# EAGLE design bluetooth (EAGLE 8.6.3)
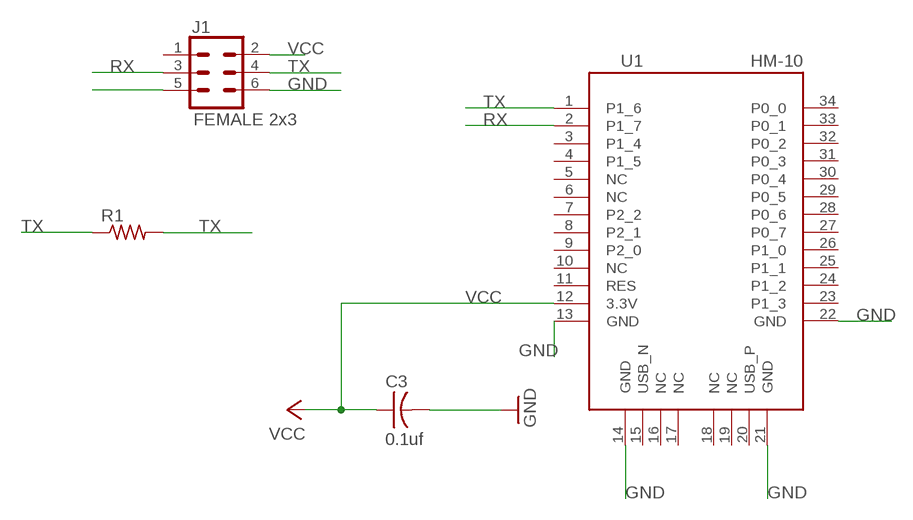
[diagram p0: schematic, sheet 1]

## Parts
C3  0.1uf  CAP-US1206FAB  [C1206FAB]
J1  FEMALE 2x3  CONN_03X2FEMALE  [2X3]
R1  RES-US1206FAB  [R1206FAB]
U1  HM-10  [HM-10]

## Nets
GND: C3.2 J1.6 U1.13(GND) U1.14(GND) U1.21(GND) U1.22(GND)
N$2: J1.5
RX: J1.3 U1.2(P1_7)
TX: J1.4 R1.1 R1.2 U1.1(P1_6)
VCC: C3.1 J1.2 U1.12(3.3V)
Unconnected: J1.1 U1.3(P1_4) U1.4(P1_5) U1.5(NC) U1.6(NC) U1.7(P2_2) U1.8(P2_1) U1.9(P2_0) U1.10(NC) U1.11(RES) U1.15(USB_N) U1.16(NC) U1.17(NC) U1.18(NC) U1.19(NC) U1.20(USB_P) U1.23(P1_3) U1.24(P1_2) U1.25(P1_1) U1.26(P1_0) U1.27(P0_7) U1.28(P0_6) U1.29(P0_5) U1.30(P0_4) U1.31(P0_3) U1.32(P0_2) U1.33(P0_1) U1.34(P0_0)

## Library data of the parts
C3 = private:CAP-US
J1 = private:CONN_03X2: Multi connection point. Often used as Generic Header-pin footprint for 0.1 inch spaced/style header connections You can populate with any combo of single row headers, but if you'd like an exact match, check these: Header - 2x3 (Male, 0.1") (PRT-12807) Header - 2x3 (Female, 0.1") (PRT-13010) 2x3 Pin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; PROD_ID: CONN-11566
R1 = private:RES-US: Resistor (US Symbol)
U1 = private:HM-10

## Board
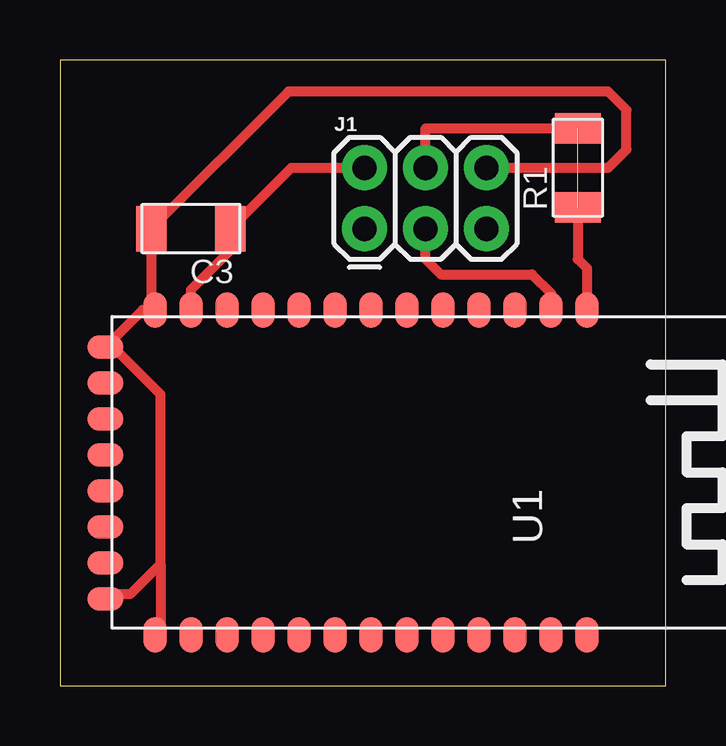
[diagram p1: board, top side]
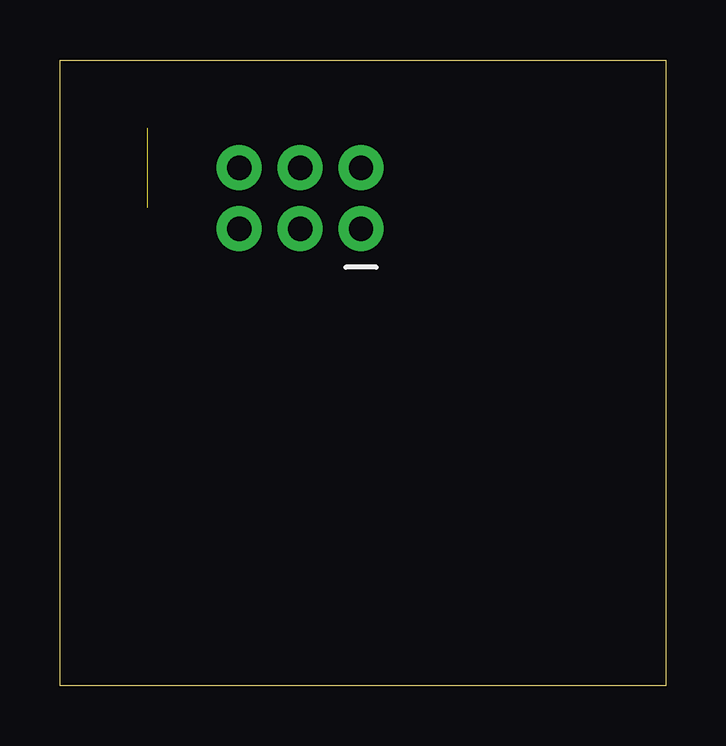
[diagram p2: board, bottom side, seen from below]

Size 25.25 x 26.09 mm. Coordinates in mm from the lower left corner, seen from the top.
Outline: 0,0 25.25,0 25.25,26.09 0,26.09 0,0
Copper layers (1*16): Top 0.035mm / dielectric 1.5mm / Bottom 0.035mm
Design rules "default *": minimum track width 15mil, minimum drill 0.79mm, track to track 0.4mm, track to pad 0.4mm, pad to pad 0.4mm, via to via 0.4mm, smd to smd 0.4mm, copper to edge 40mil, drill to drill 6mil, minimum pad ring 10mil, minimum via ring 8mil, stop-mask expansion 4mil, vias tented up to drill 0mil, thermal gap 10mil

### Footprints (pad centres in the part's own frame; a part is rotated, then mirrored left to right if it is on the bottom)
C1206FAB = smd 1.27 x 1.905: 1 -1.651,0; 2 1.651,0
2X3 = drill 1.016 pad 1.88: 1 0,0; 2 0,2.54; 3 2.54,0; 4 2.54,2.54; 5 5.08,0; 6 5.08,2.54
R1206FAB = smd 1.27 x 1.905: 1 -1.651,0; 2 1.651,0
HM-10 = smd 1.5 x 1: 1 -6.77,6.35; 2 -6.77,4.85; 3 -6.77,3.35; 4 -6.77,1.85; 5 -6.77,0.35; 6 -6.77,-1.15; 7 -6.77,-2.65; 8 -6.77,-4.15; 9 -6.77,-5.65; 10 -6.77,-7.15; 11 -6.77,-8.65; 12 -6.77,-10.15; 13 -6.77,-11.65; 22 6.77,-11.65; 23 6.77,-10.15; 24 6.77,-8.65; 25 6.77,-7.15; 26 6.77,-5.65; 27 6.77,-4.15; 28 6.77,-2.65; 29 6.77,-1.15; 30 6.77,0.35; 31 6.77,1.85; 32 6.77,3.35; 33 6.77,4.85; 34 6.77,6.35 | smd 1 x 1.5: 14 -5.23,-13.72; 15 -3.73,-13.72; 16 -2.23,-13.72; 17 -0.73,-13.72; 18 0.77,-13.72; 19 2.27,-13.72; 20 3.77,-13.72; 21 5.27,-13.72

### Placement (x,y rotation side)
C3  5.46,19.05 180 top
J1  12.7,19.05 0 top
R1  21.59,21.59 90 top
U1  15.62,8.89 270 top

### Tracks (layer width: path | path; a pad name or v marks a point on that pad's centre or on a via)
GND
  Top 0.406: 4.19,5.08 4.19,12.14 2.21,14.12 U1.14 3.44,15.66 U1.13 3.81,15.82 C3.2 9.53,24.77 22.86,24.77 23.62,24 23.62,22.35 22.86,21.59 J1.6 | 4.19,5.08 2.92,3.81 2.09,3.81 U1.21 | 4.19,5.08 4.19,2.34 U1.22
RX
  Top 0.406: U1.2 20.47,16.36 19.68,17.14 15.88,17.14 15.24,17.78 J1.3
TX  (1 unrouted)
  Top 0.406: U1.1 21.97,17.4 21.59,17.78 R1.1 | R1.2 15.24,23.24 J1.4
VCC
  Top 0.406: U1.12 5.46,16.51 7.11,18.16 C3.1 9.65,21.59 J1.2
